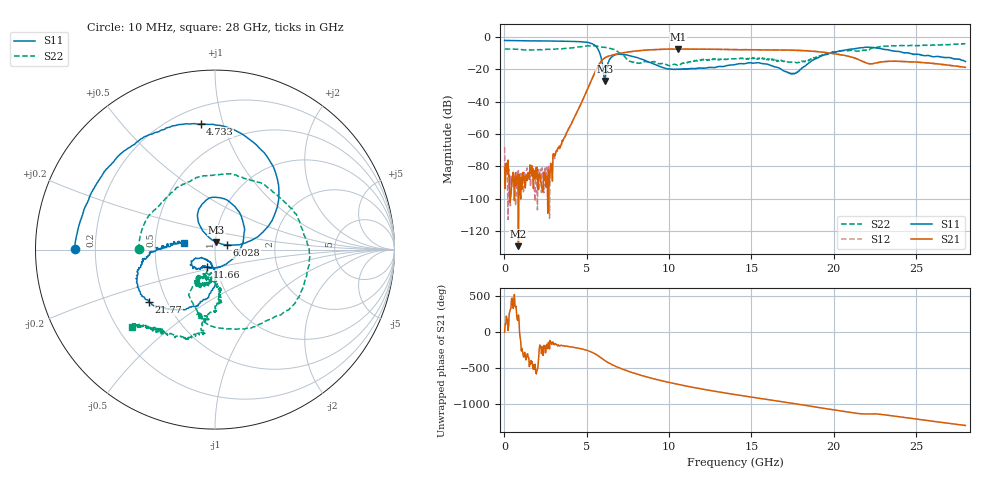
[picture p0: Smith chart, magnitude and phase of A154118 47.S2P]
!  2-Port S-parameters saved by WinCal
! VAR MeasName=S-Parameters (CALIBRATED_DATA) read from VNA (N5230A)
! VAR MeasDate=2015-9-10 14:38:07
! VAR NAME=A154118 47
! VAR FILENAME=A154118 47.S2P
! VAR DATE=2015-9-10 14:38:07
! VAR PHYS_PORTS=1,2
# Hz S DB R 50
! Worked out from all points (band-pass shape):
!   801 points, 10 MHz to 28 GHz, reference 50 ohm
!   highest |S21| = -7.45 dB at 10.54 GHz (marker M1); lowest = -129.4 dB at 849.7 MHz (marker M2)
!   |S21| within 3 dB of the highest: 6.855 GHz to 20.1 GHz (13.25 GHz wide, 98.3 % of centre)
!   lowest |S11| = -27.3 dB at 6.098 GHz (marker M3), VSWR 1.09, Z = 50.7 + j4.32 ohm
!   |S11| at or under -10 dB: 5.79 GHz to 19.77 GHz (13.98 GHz wide, 109 % of centre); 24.57 GHz to end of sweep
!   |S22| runs from -17.8 to -4.0 dB; largest |S21 - S12| = 0.0068
!   S11 on the Smith chart (normalised r, x): 10 MHz: 0.12, +0.00; 4.733 GHz: 0.30, +0.84; 6.028 GHz: 1.14, +0.06; 11.66 GHz: 0.90, -0.18; 21.77 GHz: 0.40, -0.30; 28 GHz: 0.71, +0.06
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1e7  -2.15 179.7  -80.52 -7.4  -68.19 98.4  -7.49 179.8
1.849375e8  -2.16 177.2  -84.75 161.3  -90.99 16.7  -7.43 174.3
8.497e8  -2.30 168.4  -129.42 -126.7  -82.60 84.2  -7.65 153.7
2.774012e9  -2.49 142.1  -83.13 -120.0  -84.42 161.2  -7.66 97.3
4.698325e9  -3.02 98.1  -40.18 120.6  -40.11 120.1  -5.99 11.8
4.733312e9  -3.04 96.5  -39.33 118.4  -39.28 118.2  -5.99 9.6
5.608e9  -6.41 41.8  -19.54 38.5  -19.52 38.5  -5.59 -40.3
6.02785e9  -23.06 21.2  -13.44 -29.1  -13.46 -29.3  -6.36 -63.7
6.097825e9  -27.25 78.9  -12.94 -40.0  -12.95 -40.1  -6.37 -66.1
6.58765e9  -11.83 107.6  -11.09 -103.6  -11.11 -103.9  -7.45 -93.9
7.532312e9  -11.37 68.8  -9.23 169.7  -9.21 169.7  -14.54 -123.4
8.476975e9  -14.20 32.9  -8.20 102.4  -8.22 102.3  -15.14 -106.2
9.351662e9  -17.88 -12.1  -7.73 49.6  -7.68 49.5  -16.50 -114.6
1.054124e10  -19.82 -75.7  -7.45 -12.0  -7.43 -12.4  -17.43 -98.9
1.166084e10  -19.50 -114.3  -7.51 -62.2  -7.50 -62.7  -14.46 -98.6
1.4005e10  -17.11 -131.2  -7.81 -153.2  -7.80 -153.7  -13.52 -112.4
1.557944e10  -16.26 -148.6  -7.99 151.3  -8.00 150.4  -12.83 -117.6
1.753874e10  -22.46 -121.8  -8.18 83.4  -8.24 82.7  -15.55 -108.4
1.869332e10  -14.53 -88.9  -8.78 41.2  -8.80 40.8  -13.00 -83.9
2.177222e10  -6.56 -141.6  -15.20 -62.2  -15.23 -63.2  -8.20 -101.3
2.334666e10  -8.07 -172.5  -15.01 -82.8  -15.04 -83.7  -5.69 -111.4
2.8e10  -15.17 167.3  -18.78 137.5  -18.79 137.0  -4.01 -136.9
